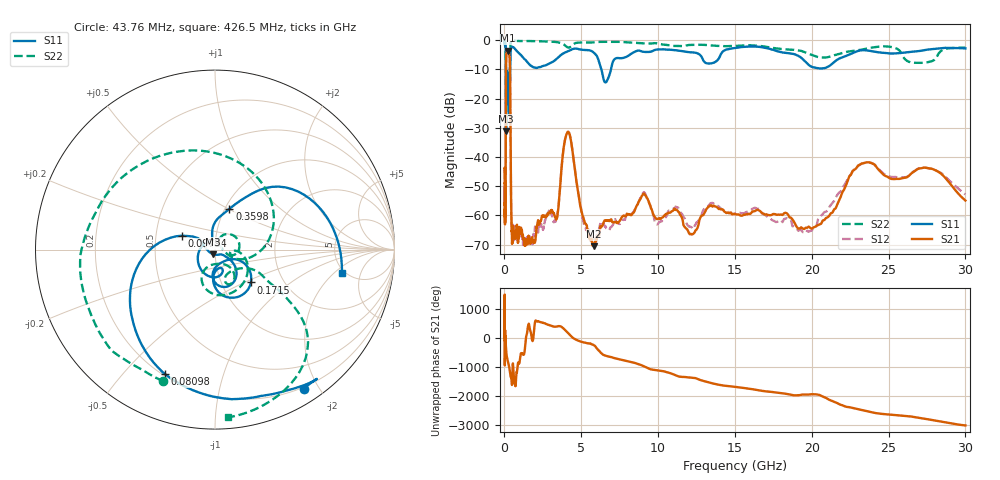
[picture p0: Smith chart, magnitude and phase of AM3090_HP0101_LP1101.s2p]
! Date/Time: Thu, Feb 28, 2019 1:59 PM
! Network Analyzer: Agilent Technologies E8364B Rev: A.07.50.67
! Sweep from 0.010 to 30.000 GHz, 1601 Points, Sweep Type: LOG
! Power Supply: 5.023 V, 0.002 A
# Hz S DB R 50
!freq MagS11 AngS11 MagS21 AngS21 MagS12 AngS12 MagS22 AngS22
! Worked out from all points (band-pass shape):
!   1601 points, 10 MHz to 30 GHz, reference 50 ohm
!   highest |S21| = -3.59 dB at 236.3 MHz (marker M1); lowest = -70.5 dB at 5.841 GHz (marker M2)
!   |S21| within 3 dB of the highest: 109.1 MHz to 343.9 MHz (234.8 MHz wide, 104 % of centre)
!   lowest |S11| = -31.2 dB at 105.1 MHz (marker M3), VSWR 1.06, Z = 49 - j2.54 ohm
!   |S11| at or under -10 dB: 95.93 MHz to 370.1 MHz (274.1 MHz wide, 118 % of centre); 6.308 GHz to 6.931 GHz (622.8 MHz wide, 9.41 % of centre)
!   |S22| runs from -29.2 to -0.1 dB; largest |S21 - S12| = 0.011
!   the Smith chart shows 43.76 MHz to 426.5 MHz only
!   S11 on the Smith chart (normalised r, x): 43.76 MHz: 0.18, -1.81; 80.98 MHz: 0.21, -0.65; 97.94 MHz: 0.68, +0.11; 171.5 MHz: 1.38, -0.54; 359.8 MHz: 1.05, +0.51; 426.5 MHz: 4.67, -2.56
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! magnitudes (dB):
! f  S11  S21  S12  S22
! 10 MHz  -0.2  -43.8  -44.7  -0.7
! 38.04 MHz  -0.5  -58.9  -59.7  -1.6
! 43.76 MHz  -0.7  -58.2  -59.8  -2.1
! 80.98 MHz  -2.5  -49.3  -47.8  -4.6
! 97.94 MHz  -13.9  -14.6  -14.5  -13.9
! 105.1 MHz  -31.2  -8.0  -8.0  -28.7
! 120.2 MHz  -13.5  -5.1  -5.1  -17.9
! 144.7 MHz  -21.8  -3.9  -3.9  -21.3
! 171.5 MHz  -11.3  -3.7  -3.7  -13.5
! 236.3 MHz  -19.5  -3.6  -3.6  -18.2
! 319 MHz  -25.2  -5.0  -4.9  -16.3
! 359.8 MHz  -12.4  -9.2  -9.2  -8.2
! 426.5 MHz  -2.9  -51.8  -54.5  -0.6
! 550.5 MHz  -2.4  -63.7  -64.1  -0.2
! 2.084 GHz  -9.5  -64.2  -65.1  -0.4
! 3.335 GHz  -6.7  -61.1  -61.9  -0.6
! 4.136 GHz  -3.8  -31.4  -31.3  -2.5
! 5.841 GHz  -4.4  -70.5  -67.2  -0.7
! 7.926 GHz  -5.7  -60.1  -60.1  -0.7
! 19.51 GHz  -7.0  -64.6  -65.8  -4.0
! 23.59 GHz  -3.5  -41.8  -41.8  -2.9
! 30 GHz  -2.8  -54.9  -52.8  -2.6
